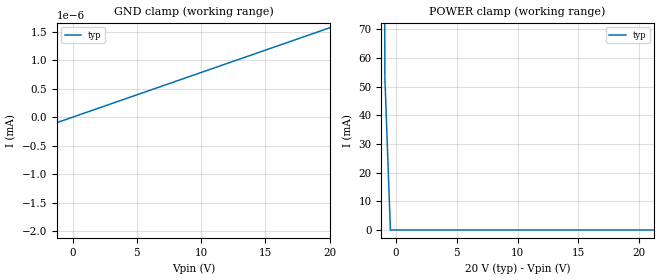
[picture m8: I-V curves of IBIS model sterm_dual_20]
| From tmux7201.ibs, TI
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| sterm_dual_20
[Model]   sterm_dual_20
Model_type   Terminator
|   typ   min   max
C_comp   4.014581e-11   NA   NA
[Voltage Range]   20   NA   NA
[Temperature Range]   27   NA   NA
[Power Clamp Reference]   20   NA   NA
[GND Clamp Reference]   0   NA   NA
[GND Clamp]
|   Voltage   I(typ)   I(min)   I(max)
-25V      -10.51A    NA         NA
-20.45V   -42.59nA   NA         NA
-20V      -1.566nA   NA         NA
20V       1.565nA    NA         NA
[POWER Clamp]
|   Voltage   I(typ)   I(min)   I(max)
-5V       13.28A     NA         NA
-1.364V   841.5mA    NA         NA
-909.1mV  53.34mA    NA         NA
-454.5mV  32.71nA    NA         NA
40V       -1.566nA   NA         NA
